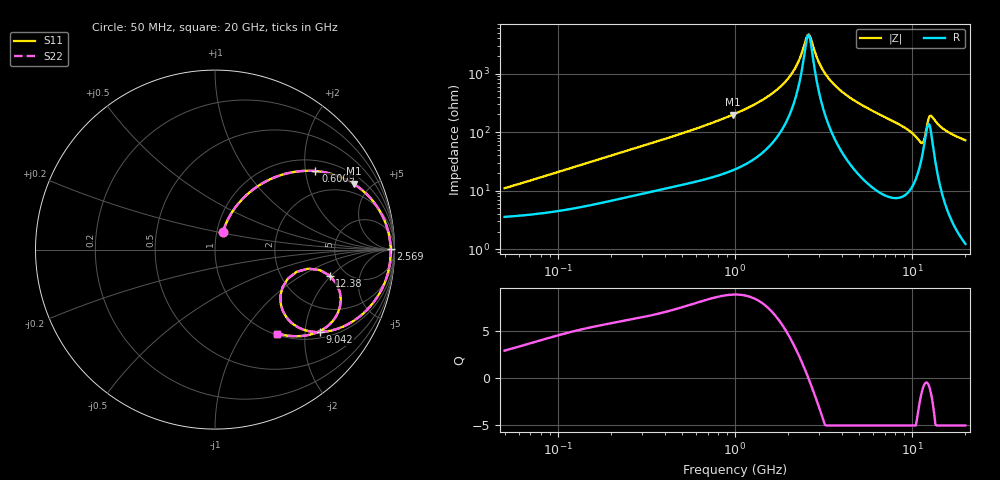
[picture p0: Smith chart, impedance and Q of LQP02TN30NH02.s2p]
!Murata Part Number: LQP02TN30NH02
!These Parameters are Measured in Series Mode Connection
!  o--[Z]--o
!Port1  Port2
!  o-------o
!Freq. Start=50[MHz] Stop=20[GHz], 401[Steps]
# Hz S RI R 50
!Freq.(Hz) S11(Real) S11(Imag) S21(Real) S21(Imag) S12(Real) S12(Imag) S22(Real) S22(Imag)
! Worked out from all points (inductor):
!   401 points, 50 MHz to 20 GHz, reference 50 ohm
!   read as one part in series: L = 32.8 nH near 52.3 MHz
!   highest Q = 8.85 at 970.5 MHz (marker M1), where L = 32.3 nH
!   self-resonance near 2.569 GHz
!   S11 on the Smith chart (normalised r, x): 50 MHz: 1.07, +0.21; 600.9 MHz: 1.28, +2.27; 2.569 GHz: 89, +20; 9.042 GHz: 1.16, -2.40; 12.38 GHz: 3.77, -1.92; 20 GHz: 1.02, -1.45
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5e7  0.0441 0.0961  0.9559 -0.0961  0.9559 -0.0961  0.0441 0.0961
1.364002e8  0.1099 0.2307  0.8901 -0.2307  0.8901 -0.2307  0.1099 0.2307
3.721004e8  0.3547 0.4109  0.6453 -0.4109  0.6453 -0.4109  0.3547 0.4109
6.009314e8  0.5591 0.4376  0.4409 -0.4376  0.4409 -0.4376  0.5591 0.4376
9.70487e8  0.7723 0.3667  0.2277 -0.3667  0.2277 -0.3667  0.7723 0.3667
1e9  0.7841 0.3588  0.2159 -0.3588  0.2159 -0.3588  0.7841 0.3588
1.432596e9  0.9009 0.2422  0.0991 -0.2422  0.0991 -0.2422  0.9009 0.2422
1.875929e9  0.9542 0.1366  0.0458 -0.1366  0.0458 -0.1366  0.9542 0.1366
2.211938e9  0.972 0.0683  0.028 -0.0683  0.028 -0.0683  0.972 0.0683
2.569357e9  0.9788 0.00478  0.0212 -0.00478  0.0212 -0.00478  0.9788 0.00478
2.728004e9  0.979 -0.0209  0.021 0.0209  0.021 0.0209  0.979 -0.0209
3.121702e9  0.9742 -0.079  0.0258 0.079  0.0258 0.079  0.9742 -0.079
3.736399e9  0.9557 -0.1568  0.0443 0.1568  0.0443 0.1568  0.9557 -0.1568
7.442007e9  0.7231 -0.4246  0.2769 0.4246  0.2769 0.4246  0.7231 -0.4246
9.041845e9  0.5855 -0.4596  0.4145 0.4596  0.4145 0.4596  0.5855 -0.4596
1.034674e10  0.4445 -0.4217  0.5555 0.4217  0.5555 0.4217  0.4445 -0.4217
1.115139e10  0.3657 -0.2998  0.6343 0.2998  0.6343 0.2998  0.3657 -0.2998
1.183995e10  0.456 -0.1233  0.544 0.1233  0.544 0.1233  0.456 -0.1233
1.238412e10  0.6395 -0.1451  0.3605 0.1451  0.3605 0.1451  0.6395 -0.1451
1.314879e10  0.6958 -0.32  0.3042 0.32  0.3042 0.32  0.6958 -0.32
1.438523e10  0.604 -0.4431  0.396 0.4431  0.396 0.4431  0.604 -0.4431
2e10  0.347 -0.4676  0.653 0.4676  0.653 0.4676  0.347 -0.4676
